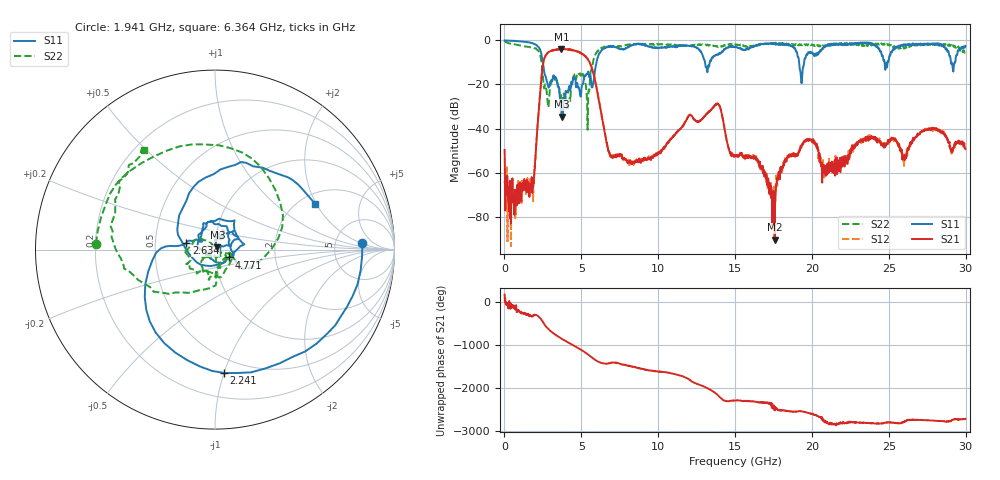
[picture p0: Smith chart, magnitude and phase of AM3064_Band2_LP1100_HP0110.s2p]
# Hz S DB R 50.0
!freq dBS11 angS11 dBS21 angS21 dBS12 angS12 dBS22 angS22
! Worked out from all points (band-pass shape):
!   1600 points, 10 MHz to 29.98 GHz, reference 50 ohm
!   highest |S21| = -3.85 dB at 3.703 GHz (marker M1); lowest = -90.5 dB at 17.57 GHz (marker M2)
!   |S21| within 3 dB of the highest: 2.678 GHz to 5.184 GHz (2.506 GHz wide, 63.8 % of centre)
!   lowest |S11| = -34.5 dB at 3.721 GHz (marker M3), VSWR 1.04, Z = 51.3 + j1.38 ohm
!   |S11| at or under -10 dB: 2.492 GHz to 5.989 GHz (3.497 GHz wide, 82.5 % of centre); 13.05 GHz to 13.35 GHz (305.1 MHz wide, 2.31 % of centre); 19.17 GHz to 19.49 GHz (325.9 MHz wide, 1.69 % of centre)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
!   |S22| runs from -40.5 to -0.3 dB; largest |S21 - S12| = 0.021
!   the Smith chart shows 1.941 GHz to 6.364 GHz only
!   S11 on the Smith chart (normalised r, x): 1.941 GHz: 10, +2; 2.241 GHz: 0.38, -1.00; 2.634 GHz: 0.72, +0.06; 4.771 GHz: 1.17, -0.10; 6.364 GHz: 2.39, +1.96
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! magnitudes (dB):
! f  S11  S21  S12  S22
! 10 MHz  0.0  -49.7  -63.9  -0.3
! 684.8 MHz  -0.2  -67.7  -70.3  -1.8
! 1.941 GHz  -1.7  -61.3  -59.5  -3.5
! 2.241 GHz  -3.2  -31.0  -30.9  -5.0
! 2.634 GHz  -15.7  -7.5  -7.5  -20.2
! 3.703 GHz  -31.4  -3.9  -4.0  -25.2
! 3.721 GHz  -34.5  -4.0  -3.8  -25.3
! 4.771 GHz  -20.9  -5.2  -5.1  -16.1
! 5.015 GHz  -21.5  -6.0  -5.9  -16.5
! 5.427 GHz  -14.4  -8.7  -8.6  -31.9
! 6.364 GHz  -4.2  -35.8  -35.8  -3.4
! 6.983 GHz  -2.8  -53.1  -52.9  -2.6
! 10 GHz  -3.4  -50.8  -51.3  -1.8
! 13.82 GHz  -6.3  -28.7  -28.7  -2.5
! 15 GHz  -2.8  -52.4  -52.5  -1.9
! 16.39 GHz  -2.2  -53.4  -53.8  -2.5
! 17.57 GHz  -1.4  -90.5  -70.6  -1.3
! 19.33 GHz  -19.4  -47.4  -47.8  -2.2
! 19.99 GHz  -5.4  -45.5  -45.7  -1.8
! 20.82 GHz  -2.9  -59.5  -56.9  -2.3
! 25 GHz  -9.0  -45.8  -45.7  -1.8
! 29.98 GHz  -2.5  -49.3  -49.2  -4.6
